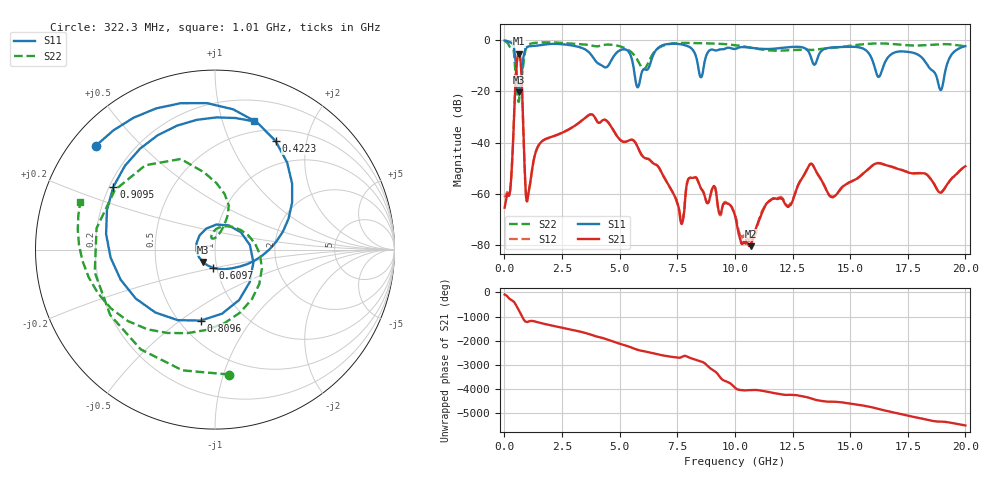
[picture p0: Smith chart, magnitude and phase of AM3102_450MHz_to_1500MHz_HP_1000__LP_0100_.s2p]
!Agilent Technologies,E8364B,MY43040894,A.07.50.67
!Agilent E8364B: A.07.50.67
!Date: Thursday, January 11, 2018 05:57:17
!Correction: S11(Full 2 Port(1,2))
!S21(Full 2 Port(1,2))
!S12(Full 2 Port(1,2))
!S22(Full 2 Port(1,2))
!S2P File: Measurements: S11, S21, S12, S22:
# Hz S  dB  R 50
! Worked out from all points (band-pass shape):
!   1601 points, 10 MHz to 20 GHz, reference 50 ohm
!   highest |S21| = -5.18 dB at 622.2 MHz (marker M1); lowest = -80.6 dB at 10.7 GHz (marker M2)
!   |S21| within 3 dB of the highest: 546.2 MHz to 703.5 MHz (157.3 MHz wide, 25.2 % of centre)
!   lowest |S11| = -20.3 dB at 634.7 MHz (marker M3), VSWR 1.21, Z = 43.3 - j6.06 ohm
!   |S11| at or under -10 dB: 5.593 GHz to 6.296 GHz (702.5 MHz wide, 11.8 % of centre); 16.05 GHz to 16.45 GHz (401.5 MHz wide, 2.47 % of centre); 18.37 GHz to 19.18 GHz (812 MHz wide, 4.32 % of centre)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
!   |S22| runs from -24.2 to -0.3 dB; largest |S21 - S12| = 0.002
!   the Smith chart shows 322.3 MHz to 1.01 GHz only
!   S11 on the Smith chart (normalised r, x): 322.3 MHz: 0.07, +0.37; 422.3 MHz: 0.65, +1.50; 609.7 MHz: 0.95, -0.19; 809.6 MHz: 0.63, -0.60; 909.5 MHz: 0.22, +0.27; 1.01 GHz: 0.39, +1.27
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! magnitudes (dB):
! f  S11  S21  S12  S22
! 10 MHz  -0.1  -65.5  -61.5  -0.3
! 322.3 MHz  -1.1  -50.0  -49.9  -3.1
! 422.3 MHz  -3.2  -28.5  -28.6  -5.4
! 609.7 MHz  -19.9  -5.2  -5.2  -24.0
! 622.2 MHz  -20.2  -5.2  -5.2  -24.2
! 634.7 MHz  -20.3  -5.3  -5.3  -23.8
! 809.6 MHz  -7.9  -31.7  -31.9  -10.1
! 909.5 MHz  -3.5  -56.3  -56.4  -4.0
! 1.01 GHz  -2.5  -61.7  -61.7  -2.0
! 1.534 GHz  -1.9  -40.4  -40.4  -0.9
! 3.346 GHz  -2.9  -31.5  -31.5  -1.6
! 5.782 GHz  -18.4  -41.8  -41.8  -7.8
! 6.682 GHz  -2.9  -49.5  -49.5  -3.1
! 7.681 GHz  -1.6  -71.9  -70.8  -1.1
! 8.218 GHz  -4.3  -53.8  -53.7  -1.1
! 10.01 GHz  -3.4  -68.7  -68.5  -1.9
! 10.7 GHz  -2.9  -80.6  -77.5  -2.9
! 13.34 GHz  -7.8  -48.4  -48.4  -3.8
! 14.22 GHz  -2.8  -61.3  -61.4  -3.0
! 16.68 GHz  -6.3  -49.2  -49.1  -1.4
! 18.93 GHz  -19.5  -59.6  -59.5  -1.5
! 20 GHz  -2.3  -49.3  -49.3  -2.3
